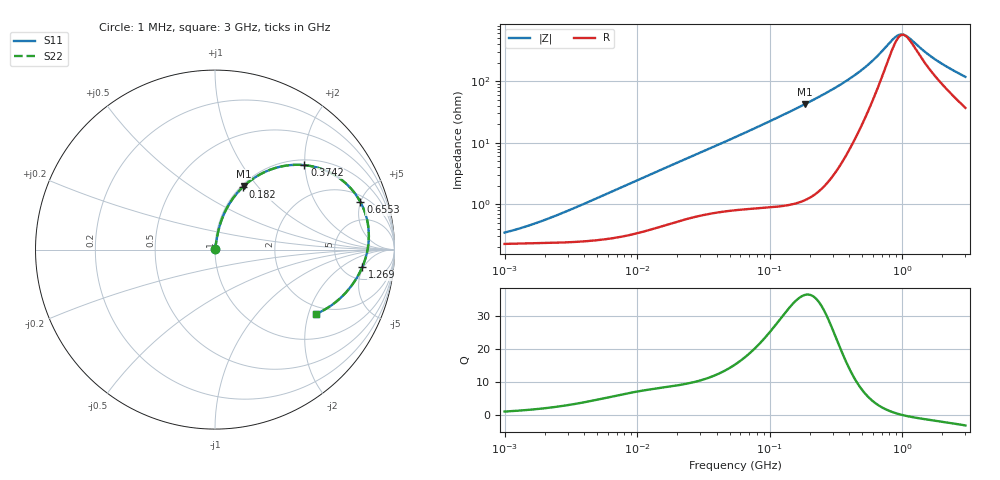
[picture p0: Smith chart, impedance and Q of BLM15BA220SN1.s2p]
! BLM15BA220SN1
# Hz S RI R 50
!Freq.(Hz) S11(Real) S11(Imag) S21(Real) S21(Imag) S12(Real) S12(Imag) S22(Real) S22(Imag)
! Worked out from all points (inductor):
!   401 points, 1 MHz to 3 GHz, reference 50 ohm
!   read as one part in series: L = 39.5 nH near 2.947 MHz
!   highest Q = 36.4 at 185.7 MHz (marker M1), where L = 36.6 nH
!   self-resonance near 1.032 GHz
!   S11 on the Smith chart (normalised r, x): 1 MHz: 1.00, +0.01; 182 MHz: 1.02, +0.84; 374.2 MHz: 1.12, +1.99; 655.3 MHz: 2.58, +4.99; 1.269 GHz: 7.60, -4.68; 3 GHz: 1.74, -2.24
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1000000  0.00227 0.00262  0.9977 -0.00262  0.9977 -0.00262  0.00227 0.00262
1786863  0.00235 0.0045  0.9977 -0.0045  0.9977 -0.0045  0.00235 0.0045
3823119  0.00257 0.00945  0.9974 -0.00945  0.9974 -0.00945  0.00257 0.00945
1.461624e7  0.00544 0.0347  0.9946 -0.0347  0.9946 -0.0347  0.00544 0.0347
5.477226e7  0.0224 0.119  0.9776 -0.119  0.9776 -0.119  0.0224 0.119
1.103592e8  0.065 0.2288  0.935 -0.2288  0.935 -0.2288  0.065 0.2288
1.820241e8  0.1557 0.349  0.8443 -0.349  0.8443 -0.349  0.1557 0.349
1.857042e8  0.1612 0.3543  0.8388 -0.3543  0.8388 -0.3543  0.1612 0.3543
2.094008e8  0.199 0.3857  0.801 -0.3857  0.801 -0.3857  0.199 0.3857
2.771263e8  0.3195 0.4494  0.6805 -0.4494  0.6805 -0.4494  0.3195 0.4494
3.741707e8  0.4985 0.4706  0.5015 -0.4706  0.5015 -0.4706  0.4985 0.4706
5.051982e8  0.6911 0.3994  0.3089 -0.3994  0.3089 -0.3994  0.6911 0.3994
6.553423e8  0.8104 0.2648  0.1896 -0.2648  0.1896 -0.2648  0.8104 0.2648
8.005644e8  0.8518 0.1433  0.1482 -0.1433  0.1482 -0.1433  0.8518 0.1433
9.0272e8  0.8573 0.0727  0.1427 -0.0727  0.1427 -0.0727  0.8573 0.0727
9.977393e8  0.8531 0.0177  0.1469 -0.0177  0.1469 -0.0177  0.8531 0.0177
1.10276e9  0.8428 -0.0332  0.1572 0.0332  0.1572 0.0332  0.8428 -0.0332
1.268618e9  0.8206 -0.0976  0.1794 0.0976  0.1794 0.0976  0.8206 -0.0976
1.519029e9  0.7822 -0.1699  0.2178 0.1699  0.2178 0.1699  0.7822 -0.1699
1.855641e9  0.7296 -0.2388  0.2704 0.2388  0.2704 0.2388  0.7296 -0.2388
2.359433e9  0.6532 -0.3072  0.3468 0.3072  0.3468 0.3072  0.6532 -0.3072
3e9  0.5631 -0.358  0.4369 0.358  0.4369 0.358  0.5631 -0.358
